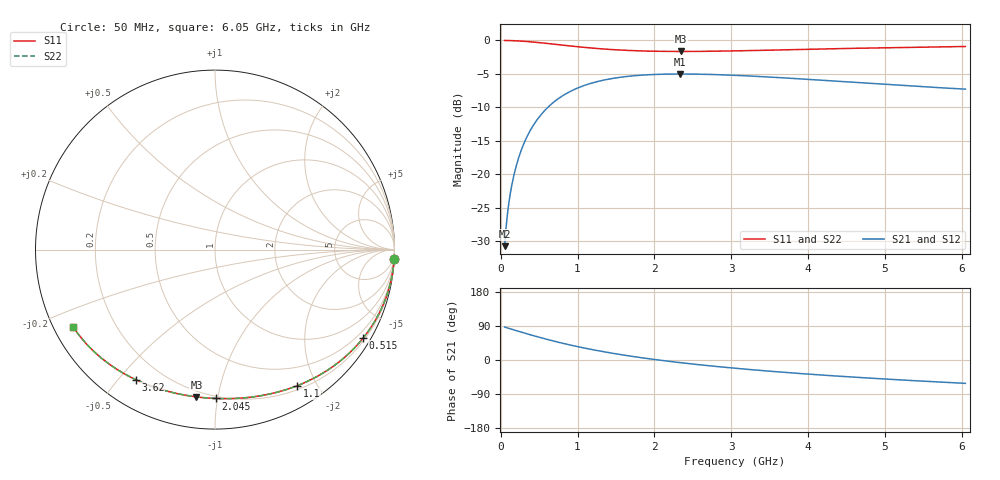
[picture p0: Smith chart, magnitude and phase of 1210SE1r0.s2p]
! AVX Thin Film Operation		Date: August 2001
! Description: Accu-P® Series, Thin Film, SMD, RF Capacitor
! Part Number: 12101J1R0ABT
! 50 MHz  -  6.05 GHz
! Serial Measurements
# mhz S db R 50
!	S11		S21		S12		S22
!	dB	Phase	dB	Phase	dB	Phase	dB	Phase
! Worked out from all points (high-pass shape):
!   401 points, 50 MHz to 6.05 GHz, reference 50 ohm
!   highest |S21| = -5.01 dB at 2.33 GHz (marker M1); lowest = -30.7 dB at 50 MHz (marker M2)
!   |S21| within 3 dB of the highest: 842 MHz to end of sweep
!   lowest |S11| = -1.6 dB at 2.345 GHz (marker M3), VSWR 10.57, Z = 8.35 - j43.4 ohm
!   |S11| at or under -10 dB: nowhere
!   |S22| runs from -1.6 to 0.0 dB; largest |S21 - S12| = 0
!   S11 on the Smith chart (normalised r, x): 50 MHz: 0, -37; 515 MHz: 0.28, -3.61; 1.1 GHz: 0.25, -1.74; 2.045 GHz: 0.19, -0.99; 3.62 GHz: 0.11, -0.56; 6.05 GHz: 0.06, -0.25
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50  -0.00 -3.1  -30.74 86.9  -30.74 86.9  -0.00 -3.1
65  -0.01 -4.0  -28.46 86.0  -28.46 86.0  -0.01 -4.0
125  -0.02 -7.8  -22.82 82.2  -22.82 82.2  -0.02 -7.8
170  -0.04 -10.5  -20.18 79.5  -20.18 79.5  -0.04 -10.5
215  -0.07 -13.3  -18.20 76.7  -18.20 76.7  -0.07 -13.3
275  -0.11 -16.9  -16.15 73.1  -16.15 73.1  -0.11 -16.9
350  -0.17 -21.4  -14.19 68.6  -14.19 68.6  -0.17 -21.4
515  -0.34 -30.8  -11.22 59.2  -11.22 59.2  -0.34 -30.8
635  -0.49 -37.3  -9.76 52.7  -9.76 52.7  -0.49 -37.3
770  -0.66 -44.1  -8.53 45.9  -8.53 45.9  -0.66 -44.1
1055  -1.00 -57.1  -6.86 32.9  -6.86 32.9  -1.00 -57.0
1100  -1.05 -58.9  -6.68 31.1  -6.68 31.1  -1.05 -58.9
1535  -1.43 -74.9  -5.54 15.1  -5.54 15.1  -1.43 -74.9
2045  -1.62 -89.8  -5.07 0.2  -5.07 0.2  -1.62 -89.8
2060  -1.62 -90.2  -5.06 -0.2  -5.06 -0.2  -1.62 -90.2
2330  -1.65 -96.8  -5.01 -6.8  -5.01 -6.8  -1.65 -96.8
2345  -1.65 -97.2  -5.01 -7.2  -5.01 -7.2  -1.65 -97.2
3050  -1.56 -111.7  -5.21 -21.7  -5.21 -21.7  -1.56 -111.7
3620  -1.42 -121.4  -5.55 -31.4  -5.55 -31.4  -1.42 -121.4
4055  -1.31 -127.9  -5.86 -38.0  -5.86 -38.0  -1.31 -127.9
5060  -1.08 -140.8  -6.61 -50.9  -6.61 -50.9  -1.08 -140.8
6050  -0.91 -151.6  -7.28 -61.7  -7.28 -61.7  -0.91 -151.6
